| IBS file for 9Meg Burst ( GS88xxxCx )
| DQ driver is programmable
| VDD or VDDQ can be either 1.8V or 2.5V or 3.3V
|  Rev 1.0: Creation
[IBIS Ver]   3.2
[File name]   gs88xxxcx.ibs
[File Rev]   1.0
[Date]   08/12/09
[Component]   GS880f18CT
[Manufacturer]   gsi technology
[Package]
| variable   typ   min   max
R_pkg   0.2   0.1   0.5
L_pkg   4nH   2nH   6nH
C_pkg   1.5pF   1pF   2pF
[Pin]   signal_name model_name  R_pin   L_pin   C_pin
 1   NC   NC
 2   NC   NC
 3   NC   NC
 4   VDDQ   POWER
 5   VSS   GND
 6   NC   NC
 7   NC   NC
 8   DQB1   Progbuf1
 9   DQB2   Progbuf1
 10   VSS   GND
 11   VDDQ   POWER
 12   DQB3   Progbuf1
 13   DQB4   Progbuf1
 14   NC   NC
 15   VDD   POWER
 16   NC   NC
 17   VSS   GND
 18   DQB5   Progbuf1
 19   DQB6   Progbuf1
 20   VDDQ   POWER
 21   VSS   GND
 22   DQB7   Progbuf1
 23   DQB8   Progbuf1
 24   DQB9   Progbuf1
 25   NC   NC
 26   VSS   GND
 27   VDDQ   POWER
 28   NC   NC
 29   NC   NC
 30   NC   NC
 31   LBO#   INBUF
 32   A5   INBUF
 33   A4   INBUF
 34   A3   INBUF
 35   A2   INBUF
 36   A1   INBUF
 37   A0   INBUF
 38   NC   NC
 39   NC   NC
 40   VSS   GND
 41   VDD   POWER
 42   NC   NC
 43   A17   INBUF
 44   A10   INBUF
 45   A11   INBUF
 46   A12   INBUF
 47   A13   INBUF
 48   A14   INBUF
 49   A15   INBUF
 50   A16   INBUF
 51   NC   NC
 52   NC   NC
 53   NC   NC
 54   VDDQ   POWER
 55   VSS   GND
 56   DQA6   Progbuf1
 57   NC   NC
 58   DQA1   Progbuf1
 59   DQA2   Progbuf1
 60   VSS   GND
 61   VDDQ   POWER
 62   DQA3   Progbuf1
 63   DQA4   Progbuf1
 64   ZZ   INBUF
 65   VDD   POWER
 66   NC   NC
 67   VSS   GND
 68   DQA5   Progbuf1
 69   DQA6   Progbuf1
 70   VDDQ   POWER
 71   VSS   GND
 72   DQA7   Progbuf1
 73   DQA8   Progbuf1
 74   DQA9   Progbuf1
 75   NC   NC
 76   VSS   GND
 77   VDDQ   POWER
 78   NC   NC
 79   NC   NC
 80   A18   INBUF
 81   A9   INBUF
 82   A8   INBUF
 83   ADV#   INBUF
 84   ADSP#   INBUF
 85   ADSC#   INBUF
 86   G#   INBUF
 87   BW#   INBUF
 88   GW#   INBUF
 89   CK   INBUF
 90   VSS   GND
 91   VDD   POWER
 92   E3#   INBUF
 93   BA#   INBUF
 94   BB#   INBUF
 95   NC   NC
 96   NC   NC
 97   E2   INBUF
 98   E1#   INBUF
 99   A7   INBUF
 100   A6   INBUF
[Component]   GS880f32CT
[Manufacturer]   gsi technology
[Package]
| variable   typ   min   max
R_pkg   0.2   0.1   0.5
L_pkg   4nH   2nH   6nH
C_pkg   1.5pF   1pF   2pF
[Pin]   signal_name model_name  R_pin   L_pin   C_pin
 1   NC   NC
 2   DQC8   Progbuf1
 3   DQC7   Progbuf1
 4   VDDQ   POWER
 5   VSS   GND
 6   DQC6   Progbuf1
 7   DQC5   Progbuf1
 8   DQC4   Progbuf1
 9   DQC3   Progbuf1
 10   VSS   GND
 11   VDDQ   POWER
 12   DQC2   Progbuf1
 13   DQC1   Progbuf1
 14   NC   NC
 15   VDD   POWER
 16   NC   NC
 17   VSS   GND
 18   DQD1   Progbuf1
 19   DQD2   Progbuf1
 20   VDDQ   POWER
 21   VSS   GND
 22   DQD3   Progbuf1
 23   DQD4   Progbuf1
 24   DQD5   Progbuf1
 25   DQD6   Progbuf1
 26   VSS   GND
 27   VDDQ   POWER
 28   DQD7   Progbuf1
 29   DQD8   Progbuf1
 30   NC   NC
 31   LBO#   INBUF
 32   A5   INBUF
 33   A4   INBUF
 34   A3   INBUF
 35   A2   INBUF
 36   A1   INBUF
 37   A0   INBUF
 38   NC   NC
 39   NC   NC
 40   VSS   GND
 41   VDD   POWER
 42   NC   NC
 43   A17   INBUF
 44   A10   INBUF
 45   A11   INBUF
 46   A12   INBUF
 47   A13   INBUF
 48   A14   INBUF
 49   A15   INBUF
 50   A16   INBUF
 51   NC   NC
 52   DQA8   Progbuf1
 53   DQA7   Progbuf1
 54   VDDQ   POWER
 55   VSS   GND
 56   DQA6   Progbuf1
 57   DQA5   Progbuf1
 58   DQA4   Progbuf1
 59   DQA3   Progbuf1
 60   VSS   GND
 61   VDDQ   POWER
 62   DQA2   Progbuf1
 63   DQA1   Progbuf1
 64   ZZ   INBUF
 65   VDD   POWER
 66   NC   NC
 67   VSS   GND
 68   DQB1   Progbuf1
 69   DQB2   Progbuf1
 70   VDDQ   POWER
 71   VSS   GND
 72   DQB3   Progbuf1
 73   DQB4   Progbuf1
 74   DQB5   Progbuf1
 75   DQB6   Progbuf1
 76   VSS   GND
 77   VDDQ   POWER
 78   DQB7   Progbuf1
 79   DQB8   Progbuf1
 80   NC   NC
 81   A9   INBUF
 82   A8   INBUF
 83   ADV#   INBUF
 84   ADSP#   INBUF
 85   ADSC#   INBUF
 86   G#   INBUF
 87   BW#   INBUF
 88   GW#   INBUF
 89   CK   INBUF
 90   VSS   GND
 91   VDD   POWER
 92   E3#   INBUF
 93   BA#   INBUF
 94   BB#   INBUF
 95   BC#   INBUF
 96   BD#   INBUF
 97   E2   INBUF
 98   E1#   INBUF
 99   A7   INBUF
 100   A6   INBUF
[Component]   GS880f36CT
[Manufacturer]   gsi technology
[Package]
| variable   typ   min   max
R_pkg   0.2   0.1   0.5
L_pkg   4nH   2nH   6nH
C_pkg   1.5pF   1pF   2pF
[Pin]   signal_name model_name  R_pin   L_pin   C_pin
 1   DQC9   Progbuf1
 2   DQC8   Progbuf1
 3   DQC7   Progbuf1
 4   VDDQ   POWER
 5   VSS   GND
 6   DQC6   Progbuf1
 7   DQC5   Progbuf1
 8   DQC4   Progbuf1
 9   DQC3   Progbuf1
 10   VSS   GND
 11   VDDQ   POWER
 12   DQC2   Progbuf1
 13   DQC1   Progbuf1
 14   NC   NC
 15   VDD   POWER
 16   NC   NC
 17   VSS   GND
 18   DQD1   Progbuf1
 19   DQD2   Progbuf1
 20   VDDQ   POWER
 21   VSS   GND
 22   DQD3   Progbuf1
 23   DQD4   Progbuf1
 24   DQD5   Progbuf1
 25   DQD6   Progbuf1
 26   VSS   GND
 27   VDDQ   POWER
 28   DQD7   Progbuf1
 29   DQD8   Progbuf1
 30   DQD9   Progbuf1
 31   LBO#   INBUF
 32   A5   INBUF
 33   A4   INBUF
 34   A3   INBUF
 35   A2   INBUF
 36   A1   INBUF
 37   A0   INBUF
 38   NC   NC
 39   NC   NC
 40   VSS   GND
 41   VDD   POWER
 42   A18   INBUF
 43   A17   INBUF
 44   A10   INBUF
 45   A11   INBUF
 46   A12   INBUF
 47   A13   INBUF
 48   A14   INBUF
 49   A15   INBUF
 50   A16   INBUF
 51   DQA9   Progbuf1
 52   DQA8   Progbuf1
 53   DQA7   Progbuf1
 54   VDDQ   POWER
 55   VSS   GND
 56   DQA6   Progbuf1
 57   DQA5   Progbuf1
 58   DQA4   Progbuf1
 59   DQA3   Progbuf1
 60   VSS   GND
 61   VDDQ   POWER
 62   DQA2   Progbuf1
 63   DQA1   Progbuf1
 64   ZZ   INBUF
 65   VDD   POWER
 66   NC   NC
 67   VSS   GND
 68   DQB1   Progbuf1
 69   DQB2   Progbuf1
 70   VDDQ   POWER
 71   VSS   GND
 72   DQB3   Progbuf1
 73   DQB4   Progbuf1
 74   DQB5   Progbuf1
 75   DQB6   Progbuf1
 76   VSS   GND
 77   VDDQ   POWER
 78   DQB7   Progbuf1
 79   DQB8   Progbuf1
 80   DQB9   Progbuf1
 81   A9   INBUF
 82   A8   INBUF
 83   ADV#   INBUF
 84   ADSP#   INBUF
 85   ADSC#   INBUF
 86   G#   INBUF
 87   BW#   INBUF
 88   GW#   INBUF
 89   CK   INBUF
 90   VSS   GND
 91   VDD   POWER
 92   E3#   INBUF
 93   BA#   INBUF
 94   BB#   INBUF
 95   BC#   INBUF
 96   BD#   INBUF
 97   E2   INBUF
 98   E1#   INBUF
 99   A7   INBUF
 100   A6   INBUF
[Component]   GS880L18CT
[Manufacturer]   gsi technology
[Package]
| variable   typ   min   max
R_pkg   0.2   0.1   0.5
L_pkg   4nH   2nH   6nH
C_pkg   1.5pF   1pF   2pF
[Pin]   signal_name model_name  R_pin   L_pin   C_pin
 1   NC   NC
 2   NC   NC
 3   NC   NC
 4   VDDQ   POWER
 5   VSS   GND
 6   NC   NC
 7   NC   NC
 8   DQB1   Progbuf1
 9   DQB2   Progbuf1
 10   VSS   GND
 11   VDDQ   POWER
 12   DQB3   Progbuf1
 13   DQB4   Progbuf1
 14   FT#   INBUF
 15   VDD   POWER
 16   NC   NC
 17   VSS   GND
 18   DQB5   Progbuf1
 19   DQB6   Progbuf1
 20   VDDQ   POWER
 21   VSS   GND
 22   DQB7   Progbuf1
 23   DQB8   Progbuf1
 24   DQB9   Progbuf1
 25   NC   NC
 26   VSS   GND
 27   VDDQ   POWER
 28   NC   NC
 29   NC   NC
 30   NC   NC
 31   LBO#   INBUF
 32   A5   INBUF
 33   A4   INBUF
 34   A3   INBUF
 35   A2   INBUF
 36   A1   INBUF
 37   A0   INBUF
 38   NC   NC
 39   NC   NC
 40   VSS   GND
 41   VDD   POWER
 42   NC   NC
 43   A17   INBUF
 44   A10   INBUF
 45   A11   INBUF
 46   A12   INBUF
 47   A13   INBUF
 48   A14   INBUF
 49   A15   INBUF
 50   A16   INBUF
 51   NC   NC
 52   NC   NC
 53   NC   NC
 54   VDDQ   POWER
 55   VSS   GND
 56   DQA6   Progbuf1
 57   NC   NC
 58   DQA1   Progbuf1
 59   DQA2   Progbuf1
 60   VSS   GND
 61   VDDQ   POWER
 62   DQA3   Progbuf1
 63   DQA4   Progbuf1
 64   ZZ   INBUF
 65   VDD   POWER
 66   NC   NC
 67   VSS   GND
 68   DQA5   Progbuf1
 69   DQA6   Progbuf1
 70   VDDQ   POWER
 71   VSS   GND
 72   DQA7   Progbuf1
 73   DQA8   Progbuf1
 74   DQA9   Progbuf1
 75   NC   NC
 76   VSS   GND
 77   VDDQ   POWER
 78   NC   NC
 79   NC   NC
 80   A18   INBUF
 81   A9   INBUF
 82   A8   INBUF
 83   ADV#   INBUF
 84   ADSP#   INBUF
 85   ADSC#   INBUF
 86   G#   INBUF
 87   BW#   INBUF
 88   GW#   INBUF
 89   CK   INBUF
 90   VSS   GND
 91   VDD   POWER
 92   E3#   INBUF
 93   BA#   INBUF
 94   BB#   INBUF
 95   NC   NC
 96   NC   NC
 97   E2   INBUF
 98   E1#   INBUF
 99   A7   INBUF
 100   A6   INBUF
[Component]   GS880l32CT
[Manufacturer]   gsi technology
[Package]
| variable   typ   min   max
R_pkg   0.2   0.1   0.5
L_pkg   4nH   2nH   6nH
C_pkg   1.5pF   1pF   2pF
[Pin]   signal_name model_name  R_pin   L_pin   C_pin
 1   NC   NC
 2   DQC8   Progbuf1
 3   DQC7   Progbuf1
 4   VDDQ   POWER
 5   VSS   GND
 6   DQC6   Progbuf1
 7   DQC5   Progbuf1
 8   DQC4   Progbuf1
 9   DQC3   Progbuf1
 10   VSS   GND
 11   VDDQ   POWER
 12   DQC2   Progbuf1
 13   DQC1   Progbuf1
 14   FT#   INBUF
 15   VDD   POWER
 16   NC   NC
 17   VSS   GND
 18   DQD1   Progbuf1
 19   DQD2   Progbuf1
 20   VDDQ   POWER
 21   VSS   GND
 22   DQD3   Progbuf1
 23   DQD4   Progbuf1
 24   DQD5   Progbuf1
 25   DQD6   Progbuf1
 26   VSS   GND
 27   VDDQ   POWER
 28   DQD7   Progbuf1
 29   DQD8   Progbuf1
 30   NC   NC
 31   LBO#   INBUF
 32   A5   INBUF
 33   A4   INBUF
 34   A3   INBUF
 35   A2   INBUF
 36   A1   INBUF
 37   A0   INBUF
 38   NC   NC
 39   NC   NC
 40   VSS   GND
 41   VDD   POWER
 42   NC   NC
 43   A17   INBUF
 44   A10   INBUF
 45   A11   INBUF
 46   A12   INBUF
 47   A13   INBUF
 48   A14   INBUF
 49   A15   INBUF
 50   A16   INBUF
 51   NC   NC
 52   DQA8   Progbuf1
 53   DQA7   Progbuf1
 54   VDDQ   POWER
 55   VSS   GND
 56   DQA6   Progbuf1
 57   DQA5   Progbuf1
 58   DQA4   Progbuf1
 59   DQA3   Progbuf1
 60   VSS   GND
 61   VDDQ   POWER
 62   DQA2   Progbuf1
 63   DQA1   Progbuf1
 64   ZZ   INBUF
 65   VDD   POWER
 66   NC   NC
 67   VSS   GND
 68   DQB1   Progbuf1
 69   DQB2   Progbuf1
 70   VDDQ   POWER
 71   VSS   GND
 72   DQB3   Progbuf1
 73   DQB4   Progbuf1
 74   DQB5   Progbuf1
 75   DQB6   Progbuf1
 76   VSS   GND
 77   VDDQ   POWER
 78   DQB7   Progbuf1
 79   DQB8   Progbuf1
 80   NC   NC
 81   A9   INBUF
 82   A8   INBUF
 83   ADV#   INBUF
 84   ADSP#   INBUF
 85   ADSC#   INBUF
 86   G#   INBUF
 87   BW#   INBUF
 88   GW#   INBUF
 89   CK   INBUF
 90   VSS   GND
 91   VDD   POWER
 92   E3#   INBUF
 93   BA#   INBUF
 94   BB#   INBUF
 95   BC#   INBUF
 96   BD#   INBUF
 97   E2   INBUF
 98   E1#   INBUF
 99   A7   INBUF
 100   A6   INBUF
[Component]   GS880L36CT
[Manufacturer]   gsi technology
[Package]
| variable   typ   min   max
R_pkg   0.2   0.1   0.5
L_pkg   4nH   2nH   6nH
C_pkg   1.5pF   1pF   2pF
[Pin]   signal_name model_name  R_pin   L_pin   C_pin
 1   DQC9   Progbuf1
 2   DQC8   Progbuf1
 3   DQC7   Progbuf1
 4   VDDQ   POWER
 5   VSS   GND
 6   DQC6   Progbuf1
 7   DQC5   Progbuf1
 8   DQC4   Progbuf1
 9   DQC3   Progbuf1
 10   VSS   GND
 11   VDDQ   POWER
 12   DQC2   Progbuf1
 13   DQC1   Progbuf1
 14   FT#   INBUF
 15   VDD   POWER
 16   NC   NC
 17   VSS   GND
 18   DQD1   Progbuf1
 19   DQD2   Progbuf1
 20   VDDQ   POWER
 21   VSS   GND
 22   DQD3   Progbuf1
 23   DQD4   Progbuf1
 24   DQD5   Progbuf1
 25   DQD6   Progbuf1
 26   VSS   GND
 27   VDDQ   POWER
 28   DQD7   Progbuf1
 29   DQD8   Progbuf1
 30   DQD9   Progbuf1
 31   LBO#   INBUF
 32   A5   INBUF
 33   A4   INBUF
 34   A3   INBUF
 35   A2   INBUF
 36   A1   INBUF
 37   A0   INBUF
 38   NC   NC
 39   NC   NC
 40   VSS   GND
 41   VDD   POWER
 42   A18   INBUF
 43   A17   INBUF
 44   A10   INBUF
 45   A11   INBUF
 46   A12   INBUF
 47   A13   INBUF
 48   A14   INBUF
 49   A15   INBUF
 50   A16   INBUF
 51   DQA9   Progbuf1
 52   DQA8   Progbuf1
 53   DQA7   Progbuf1
 54   VDDQ   POWER
 55   VSS   GND
 56   DQA6   Progbuf1
 57   DQA5   Progbuf1
 58   DQA4   Progbuf1
 59   DQA3   Progbuf1
 60   VSS   GND
 61   VDDQ   POWER
 62   DQA2   Progbuf1
 63   DQA1   Progbuf1
 64   ZZ   INBUF
 65   VDD   POWER
 66   NC   NC
 67   VSS   GND
 68   DQB1   Progbuf1
 69   DQB2   Progbuf1
 70   VDDQ   POWER
 71   VSS   GND
 72   DQB3   Progbuf1
 73   DQB4   Progbuf1
 74   DQB5   Progbuf1
 75   DQB6   Progbuf1
 76   VSS   GND
 77   VDDQ   POWER
 78   DQB7   Progbuf1
 79   DQB8   Progbuf1
 80   DQB9   Progbuf1
 81   A9   INBUF
 82   A8   INBUF
 83   ADV#   INBUF
 84   ADSP#   INBUF
 85   ADSC#   INBUF
 86   G#   INBUF
 87   BW#   INBUF
 88   GW#   INBUF
 89   CK   INBUF
 90   VSS   GND
 91   VDD   POWER
 92   E3#   INBUF
 93   BA#   INBUF
 94   BB#   INBUF
 95   BC#   INBUF
 96   BD#   INBUF
 97   E2   INBUF
 98   E1#   INBUF
 99   A7   INBUF
 100   A6   INBUF
[Component]   GS88018CT
[Manufacturer]   gsi technology
[Package]
| variable   typ   min   max
R_pkg   0.2   0.1   0.5
L_pkg   4nH   2nH   6nH
C_pkg   1.5pF   1pF   2pF
[Pin]   signal_name model_name  R_pin   L_pin   C_pin
 1   NC   NC
 2   NC   NC
 3   NC   NC
 4   VDDQ   POWER
 5   VSS   GND
 6   NC   NC
 7   NC   NC
 8   DQB1   Progbuf1
 9   DQB2   Progbuf1
 10   VSS   GND
 11   VDDQ   POWER
 12   DQB3   Progbuf1
 13   DQB4   Progbuf1
 14   FT#   INBUF
 15   VDD   POWER
 16   NC   NC
 17   VSS   GND
 18   DQB5   Progbuf1
 19   DQB6   Progbuf1
 20   VDDQ   POWER
 21   VSS   GND
 22   DQB7   Progbuf1
 23   DQB8   Progbuf1
 24   DQB9   Progbuf1
 25   NC   NC
 26   VSS   GND
 27   VDDQ   POWER
 28   NC   NC
 29   NC   NC
 30   NC   NC
 31   LBO#   INBUF
 32   A5   INBUF
 33   A4   INBUF
 34   A3   INBUF
 35   A2   INBUF
 36   A1   INBUF
 37   A0   INBUF
 38   NC   NC
 39   NC   NC
 40   VSS   GND
 41   VDD   POWER
 42   NC   NC
 43   A17   INBUF
 44   A10   INBUF
 45   A11   INBUF
 46   A12   INBUF
 47   A13   INBUF
 48   A14   INBUF
 49   A15   INBUF
 50   A16   INBUF
 51   NC   NC
 52   NC   NC
 53   NC   NC
 54   VDDQ   POWER
 55   VSS   GND
 56   DQA6   Progbuf1
 57   NC   NC
 58   DQA1   Progbuf1
 59   DQA2   Progbuf1
 60   VSS   GND
 61   VDDQ   POWER
 62   DQA3   Progbuf1
 63   DQA4   Progbuf1
 64   ZZ   INBUF
 65   VDD   POWER
 66   NC   NC
 67   VSS   GND
 68   DQA5   Progbuf1
 69   DQA6   Progbuf1
 70   VDDQ   POWER
 71   VSS   GND
 72   DQA7   Progbuf1
 73   DQA8   Progbuf1
 74   DQA9   Progbuf1
 75   NC   NC
 76   VSS   GND
 77   VDDQ   POWER
 78   NC   NC
 79   NC   NC
 80   A18   INBUF
 81   A9   INBUF
 82   A8   INBUF
 83   ADV#   INBUF
 84   ADSP#   INBUF
 85   ADSC#   INBUF
 86   G#   INBUF
 87   BW#   INBUF
 88   GW#   INBUF
 89   CK   INBUF
 90   VSS   GND
 91   VDD   POWER
 92   E3#   INBUF
 93   BA#   INBUF
 94   BB#   INBUF
 95   NC   NC
 96   NC   NC
 97   E2   INBUF
 98   E1#   INBUF
 99   A7   INBUF
 100   A6   INBUF
[Component]   GS88019CT
[Manufacturer]   gsi technology
[Package]
| variable   typ   min   max
R_pkg   0.2   0.1   0.5
L_pkg   4nH   2nH   6nH
C_pkg   1.5pF   1pF   2pF
[Pin]   signal_name model_name  R_pin   L_pin   C_pin
 1   NC   NC
 2   NC   NC
 3   NC   NC
 4   VDDQ   POWER
 5   VSS   GND
 6   NC   NC
 7   NC   NC
 8   DQB1   Progbuf1
 9   DQB2   Progbuf1
 10   VSS   GND
 11   VDDQ   POWER
 12   DQB3   Progbuf1
 13   DQB4   Progbuf1
 14   FT#   INBUF
 15   VDD   POWER
 16   NC   NC
 17   VSS   GND
 18   DQB5   Progbuf1
 19   DQB6   Progbuf1
 20   VDDQ   POWER
 21   VSS   GND
 22   DQB7   Progbuf1
 23   DQB8   Progbuf1
 24   DQB9   Progbuf1
 25   NC   NC
 26   VSS   GND
 27   VDDQ   POWER
 28   NC   NC
 29   NC   NC
 30   NC   NC
 31   LBO#   INBUF
 32   A5   INBUF
 33   A4   INBUF
 34   A3   INBUF
 35   A2   INBUF
 36   A1   INBUF
 37   A0   INBUF
 38   NC   NC
 39   NC   NC
 40   VSS   GND
 41   VDD   POWER
 42   NC   NC
 43   A17   INBUF
 44   A10   INBUF
 45   A11   INBUF
 46   A12   INBUF
 47   A13   INBUF
 48   A14   INBUF
 49   A15   INBUF
 50   A16   INBUF
 51   NC   NC
 52   NC   NC
 53   NC   NC
 54   VDDQ   POWER
 55   VSS   GND
 56   DQA6   Progbuf1
 57   NC   NC
 58   DQA1   Progbuf1
 59   DQA2   Progbuf1
 60   VSS   GND
 61   VDDQ   POWER
 62   DQA3   Progbuf1
 63   DQA4   Progbuf1
 64   ZZ   INBUF
 65   VDD   POWER
 66   NC   NC
 67   VSS   GND
 68   DQA5   Progbuf1
 69   DQA6   Progbuf1
 70   VDDQ   POWER
 71   VSS   GND
 72   DQA7   Progbuf1
 73   DQA8   Progbuf1
 74   DQA9   Progbuf1
 75   NC   NC
 76   VSS   GND
 77   VDDQ   POWER
 78   NC   NC
 79   NC   NC
 80   A18   INBUF
 81   A9   INBUF
 82   A8   INBUF
 83   ADV#   INBUF
 84   ADSP#   INBUF
 85   ADSC#   INBUF
 86   G#   INBUF
 87   BW#   INBUF
 88   GW#   INBUF
 89   CK   INBUF
 90   VSS   GND
 91   VDD   POWER
 92   E3#   INBUF
 93   BA#   INBUF
 94   BB#   INBUF
 95   NC   NC
 96   NC   NC
 97   E2   INBUF
 98   E1#   INBUF
 99   A7   INBUF
 100   A6   INBUF
[Component]   GS88032CT
[Manufacturer]   gsi technology
[Package]
| variable   typ   min   max
R_pkg   0.2   0.1   0.5
L_pkg   4nH   2nH   6nH
C_pkg   1.5pF   1pF   2pF
[Pin]   signal_name model_name  R_pin   L_pin   C_pin
 1   NC   NC
 2   DQC8   Progbuf1
 3   DQC7   Progbuf1
 4   VDDQ   POWER
 5   VSS   GND
 6   DQC6   Progbuf1
 7   DQC5   Progbuf1
 8   DQC4   Progbuf1
 9   DQC3   Progbuf1
 10   VSS   GND
 11   VDDQ   POWER
 12   DQC2   Progbuf1
 13   DQC1   Progbuf1
 14   FT#   INBUF
 15   VDD   POWER
 16   NC   NC
 17   VSS   GND
 18   DQD1   Progbuf1
 19   DQD2   Progbuf1
 20   VDDQ   POWER
 21   VSS   GND
 22   DQD3   Progbuf1
 23   DQD4   Progbuf1
 24   DQD5   Progbuf1
 25   DQD6   Progbuf1
 26   VSS   GND
 27   VDDQ   POWER
 28   DQD7   Progbuf1
 29   DQD8   Progbuf1
 30   NC   NC
 31   LBO#   INBUF
 32   A5   INBUF
 33   A4   INBUF
 34   A3   INBUF
 35   A2   INBUF
 36   A1   INBUF
 37   A0   INBUF
 38   NC   NC
 39   NC   NC
 40   VSS   GND
 41   VDD   POWER
 42   NC   NC
 43   A17   INBUF
 44   A10   INBUF
 45   A11   INBUF
 46   A12   INBUF
 47   A13   INBUF
 48   A14   INBUF
 49   A15   INBUF
 50   A16   INBUF
 51   NC   NC
 52   DQA8   Progbuf1
 53   DQA7   Progbuf1
 54   VDDQ   POWER
 55   VSS   GND
 56   DQA6   Progbuf1
 57   DQA5   Progbuf1
 58   DQA4   Progbuf1
 59   DQA3   Progbuf1
 60   VSS   GND
 61   VDDQ   POWER
 62   DQA2   Progbuf1
 63   DQA1   Progbuf1
 64   ZZ   INBUF
 65   VDD   POWER
 66   NC   NC
 67   VSS   GND
 68   DQB1   Progbuf1
 69   DQB2   Progbuf1
 70   VDDQ   POWER
 71   VSS   GND
 72   DQB3   Progbuf1
 73   DQB4   Progbuf1
 74   DQB5   Progbuf1
 75   DQB6   Progbuf1
 76   VSS   GND
 77   VDDQ   POWER
 78   DQB7   Progbuf1
 79   DQB8   Progbuf1
 80   NC   NC
 81   A9   INBUF
 82   A8   INBUF
 83   ADV#   INBUF
 84   ADSP#   INBUF
 85   ADSC#   INBUF
 86   G#   INBUF
 87   BW#   INBUF
 88   GW#   INBUF
 89   CK   INBUF
 90   VSS   GND
 91   VDD   POWER
 92   E3#   INBUF
 93   BA#   INBUF
 94   BB#   INBUF
 95   BC#   INBUF
 96   BD#   INBUF
 97   E2   INBUF
 98   E1#   INBUF
 99   A7   INBUF
 100   A6   INBUF
[Component]   GS88033CT
[Manufacturer]   gsi technology
[Package]
| variable   typ   min   max
R_pkg   0.2   0.1   0.5
L_pkg   4nH   2nH   6nH
C_pkg   1.5pF   1pF   2pF
[Pin]   signal_name model_name  R_pin   L_pin   C_pin
 1   NC   NC
 2   DQC8   Progbuf1
 3   DQC7   Progbuf1
 4   VDDQ   POWER
 5   VSS   GND
 6   DQC6   Progbuf1
 7   DQC5   Progbuf1
 8   DQC4   Progbuf1
 9   DQC3   Progbuf1
 10   VSS   GND
 11   VDDQ   POWER
 12   DQC2   Progbuf1
 13   DQC1   Progbuf1
 14   FT#   INBUF
 15   VDD   POWER
 16   NC   NC
 17   VSS   GND
 18   DQD1   Progbuf1
 19   DQD2   Progbuf1
 20   VDDQ   POWER
 21   VSS   GND
 22   DQD3   Progbuf1
 23   DQD4   Progbuf1
 24   DQD5   Progbuf1
 25   DQD6   Progbuf1
 26   VSS   GND
 27   VDDQ   POWER
 28   DQD7   Progbuf1
 29   DQD8   Progbuf1
 30   NC   NC
 31   LBO#   INBUF
 32   A5   INBUF
 33   A4   INBUF
 34   A3   INBUF
 35   A2   INBUF
 36   A1   INBUF
 37   A0   INBUF
 38   NC   NC
 39   NC   NC
 40   VSS   GND
 41   VDD   POWER
 42   NC   NC
 43   A17   INBUF
 44   A10   INBUF
 45   A11   INBUF
 46   A12   INBUF
 47   A13   INBUF
 48   A14   INBUF
 49   A15   INBUF
 50   A16   INBUF
 51   NC   NC
 52   DQA8   Progbuf1
 53   DQA7   Progbuf1
 54   VDDQ   POWER
 55   VSS   GND
 56   DQA6   Progbuf1
 57   DQA5   Progbuf1
 58   DQA4   Progbuf1
 59   DQA3   Progbuf1
 60   VSS   GND
 61   VDDQ   POWER
 62   DQA2   Progbuf1
 63   DQA1   Progbuf1
 64   ZZ   INBUF
 65   VDD   POWER
 66   NC   NC
 67   VSS   GND
 68   DQB1   Progbuf1
 69   DQB2   Progbuf1
 70   VDDQ   POWER
 71   VSS   GND
 72   DQB3   Progbuf1
 73   DQB4   Progbuf1
 74   DQB5   Progbuf1
 75   DQB6   Progbuf1
 76   VSS   GND
 77   VDDQ   POWER
 78   DQB7   Progbuf1
 79   DQB8   Progbuf1
 80   NC   NC
 81   A9   INBUF
 82   A8   INBUF
 83   ADV#   INBUF
 84   ADSP#   INBUF
 85   ADSC#   INBUF
 86   G#   INBUF
 87   BW#   INBUF
 88   GW#   INBUF
 89   CK   INBUF
 90   VSS   GND
 91   VDD   POWER
 92   E3#   INBUF
 93   BA#   INBUF
 94   BB#   INBUF
 95   BC#   INBUF
 96   BD#   INBUF
 97   E2   INBUF
 98   E1#   INBUF
 99   A7   INBUF
 100   A6   INBUF
[Component]   GS88036CT
[Manufacturer]   gsi technology
[Package]
| variable   typ   min   max
R_pkg   0.2   0.1   0.5
L_pkg   4nH   2nH   6nH
C_pkg   1.5pF   1pF   2pF
[Pin]   signal_name model_name  R_pin   L_pin   C_pin
 1   DQC9   Progbuf1
 2   DQC8   Progbuf1
 3   DQC7   Progbuf1
 4   VDDQ   POWER
 5   VSS   GND
 6   DQC6   Progbuf1
 7   DQC5   Progbuf1
 8   DQC4   Progbuf1
 9   DQC3   Progbuf1
 10   VSS   GND
 11   VDDQ   POWER
 12   DQC2   Progbuf1
 13   DQC1   Progbuf1
 14   FT#   INBUF
 15   VDD   POWER
 16   NC   NC
 17   VSS   GND
 18   DQD1   Progbuf1
 19   DQD2   Progbuf1
 20   VDDQ   POWER
 21   VSS   GND
 22   DQD3   Progbuf1
 23   DQD4   Progbuf1
 24   DQD5   Progbuf1
 25   DQD6   Progbuf1
 26   VSS   GND
 27   VDDQ   POWER
 28   DQD7   Progbuf1
 29   DQD8   Progbuf1
 30   DQD9   Progbuf1
 31   LBO#   INBUF
 32   A5   INBUF
 33   A4   INBUF
 34   A3   INBUF
 35   A2   INBUF
 36   A1   INBUF
 37   A0   INBUF
 38   NC   NC
 39   NC   NC
 40   VSS   GND
 41   VDD   POWER
 42   A18   INBUF
 43   A17   INBUF
 44   A10   INBUF
 45   A11   INBUF
 46   A12   INBUF
 47   A13   INBUF
 48   A14   INBUF
 49   A15   INBUF
 50   A16   INBUF
 51   DQA9   Progbuf1
 52   DQA8   Progbuf1
 53   DQA7   Progbuf1
 54   VDDQ   POWER
 55   VSS   GND
 56   DQA6   Progbuf1
 57   DQA5   Progbuf1
 58   DQA4   Progbuf1
 59   DQA3   Progbuf1
 60   VSS   GND
 61   VDDQ   POWER
 62   DQA2   Progbuf1
 63   DQA1   Progbuf1
 64   ZZ   INBUF
 65   VDD   POWER
 66   NC   NC
 67   VSS   GND
 68   DQB1   Progbuf1
 69   DQB2   Progbuf1
 70   VDDQ   POWER
 71   VSS   GND
 72   DQB3   Progbuf1
 73   DQB4   Progbuf1
 74   DQB5   Progbuf1
 75   DQB6   Progbuf1
 76   VSS   GND
 77   VDDQ   POWER
 78   DQB7   Progbuf1
 79   DQB8   Progbuf1
 80   DQB9   Progbuf1
 81   A9   INBUF
 82   A8   INBUF
 83   ADV#   INBUF
 84   ADSP#   INBUF
 85   ADSC#   INBUF
 86   G#   INBUF
 87   BW#   INBUF
 88   GW#   INBUF
 89   CK   INBUF
 90   VSS   GND
 91   VDD   POWER
 92   E3#   INBUF
 93   BA#   INBUF
 94   BB#   INBUF
 95   BC#   INBUF
 96   BD#   INBUF
 97   E2   INBUF
 98   E1#   INBUF
 99   A7   INBUF
 100   A6   INBUF
[Component]   GS88037CT
[Manufacturer]   gsi technology
[Package]
| variable   typ   min   max
R_pkg   0.2   0.1   0.5
L_pkg   4nH   2nH   6nH
C_pkg   1.5pF   1pF   2pF
[Pin]   signal_name model_name  R_pin   L_pin   C_pin
 1   DQC9   Progbuf1
 2   DQC8   Progbuf1
 3   DQC7   Progbuf1
 4   VDDQ   POWER
 5   VSS   GND
 6   DQC6   Progbuf1
 7   DQC5   Progbuf1
 8   DQC4   Progbuf1
 9   DQC3   Progbuf1
 10   VSS   GND
 11   VDDQ   POWER
 12   DQC2   Progbuf1
 13   DQC1   Progbuf1
 14   FT#   INBUF
 15   VDD   POWER
 16   NC   NC
 17   VSS   GND
 18   DQD1   Progbuf1
 19   DQD2   Progbuf1
 20   VDDQ   POWER
 21   VSS   GND
 22   DQD3   Progbuf1
 23   DQD4   Progbuf1
 24   DQD5   Progbuf1
 25   DQD6   Progbuf1
 26   VSS   GND
 27   VDDQ   POWER
 28   DQD7   Progbuf1
 29   DQD8   Progbuf1
 30   DQD9   Progbuf1
 31   LBO#   INBUF
 32   A5   INBUF
 33   A4   INBUF
 34   A3   INBUF
 35   A2   INBUF
 36   A1   INBUF
 37   A0   INBUF
 38   NC   NC
 39   NC   NC
 40   VSS   GND
 41   VDD   POWER
 42   A18   INBUF
 43   A17   INBUF
 44   A10   INBUF
 45   A11   INBUF
 46   A12   INBUF
 47   A13   INBUF
 48   A14   INBUF
 49   A15   INBUF
 50   A16   INBUF
 51   DQA9   Progbuf1
 52   DQA8   Progbuf1
 53   DQA7   Progbuf1
 54   VDDQ   POWER
 55   VSS   GND
 56   DQA6   Progbuf1
 57   DQA5   Progbuf1
 58   DQA4   Progbuf1
 59   DQA3   Progbuf1
 60   VSS   GND
 61   VDDQ   POWER
 62   DQA2   Progbuf1
 63   DQA1   Progbuf1
 64   ZZ   INBUF
 65   VDD   POWER
 66   NC   NC
 67   VSS   GND
 68   DQB1   Progbuf1
 69   DQB2   Progbuf1
 70   VDDQ   POWER
 71   VSS   GND
 72   DQB3   Progbuf1
 73   DQB4   Progbuf1
 74   DQB5   Progbuf1
 75   DQB6   Progbuf1
 76   VSS   GND
 77   VDDQ   POWER
 78   DQB7   Progbuf1
 79   DQB8   Progbuf1
 80   DQB9   Progbuf1
 81   A9   INBUF
 82   A8   INBUF
 83   ADV#   INBUF
 84   ADSP#   INBUF
 85   ADSC#   INBUF
 86   G#   INBUF
 87   BW#   INBUF
 88   GW#   INBUF
 89   CK   INBUF
 90   VSS   GND
 91   VDD   POWER
 92   E3#   INBUF
 93   BA#   INBUF
 94   BB#   INBUF
 95   BC#   INBUF
 96   BD#   INBUF
 97   E2   INBUF
 98   E1#   INBUF
 99   A7   INBUF
 100   A6   INBUF
[Component]   GS881E18CT
[Manufacturer]   gsi technology
[Package]
| variable   typ   min   max
R_pkg   0.2   0.1   0.5
L_pkg   4nH   2nH   6nH
C_pkg   1.5pF   1pF   2pF
[Pin]   signal_name model_name  R_pin   L_pin   C_pin
 1   NC   NC
 2   NC   NC
 3   NC   NC
 4   VDDQ   POWER
 5   VSS   GND
 6   NC   NC
 7   NC   NC
 8   DQB1   Progbuf1
 9   DQB2   Progbuf1
 10   VSS   GND
 11   VDDQ   POWER
 12   DQB3   Progbuf1
 13   DQB4   Progbuf1
 14   FT#   INBUF
 15   VDD   POWER
 16   NC   NC
 17   VSS   GND
 18   DQB5   Progbuf1
 19   DQB6   Progbuf1
 20   VDDQ   POWER
 21   VSS   GND
 22   DQB7   Progbuf1
 23   DQB8   Progbuf1
 24   DQB9   Progbuf1
 25   NC   NC
 26   VSS   GND
 27   VDDQ   POWER
 28   NC   NC
 29   NC   NC
 30   NC   NC
 31   LBO#   INBUF
 32   A5   INBUF
 33   A4   INBUF
 34   A3   INBUF
 35   A2   INBUF
 36   A1   INBUF
 37   A0   INBUF
 38   TMS   INBUF
 39   TDI   INBUF
 40   VSS   GND
 41   VDD   POWER
 42   TDO   Progbuf2
 43   TCK   INBUF
 44   A10   INBUF
 45   A11   INBUF
 46   A12   INBUF
 47   A13   INBUF
 48   A14   INBUF
 49   A15   INBUF
 50   A16   INBUF
 51   NC   NC
 52   NC   NC
 53   NC   NC
 54   VDDQ   POWER
 55   VSS   GND
 56   DQA6   Progbuf1
 57   NC   NC
 58   DQA1   Progbuf1
 59   DQA2   Progbuf1
 60   VSS   GND
 61   VDDQ   POWER
 62   DQA3   Progbuf1
 63   DQA4   Progbuf1
 64   ZZ   INBUF
 65   VDD   POWER
 66   NC   NC
 67   VSS   GND
 68   DQA5   Progbuf1
 69   DQA6   Progbuf1
 70   VDDQ   POWER
 71   VSS   GND
 72   DQA7   Progbuf1
 73   DQA8   Progbuf1
 74   DQA9   Progbuf1
 75   NC   NC
 76   VSS   GND
 77   VDDQ   POWER
 78   NC   NC
 79   NC   NC
 80   A18   INBUF
 81   A9   INBUF
 82   A8   INBUF
 83   ADV#   INBUF
 84   ADSP#   INBUF
 85   ADSC#   INBUF
 86   G#   INBUF
 87   BW#   INBUF
 88   GW#   INBUF
 89   CK   INBUF
 90   VSS   GND
 91   VDD   POWER
 92   A17   INBUF
 93   BA#   INBUF
 94   BB#   INBUF
 95   NC   NC
 96   NC   NC
 97   NC   NC
 98   E1#   INBUF
 99   A7   INBUF
 100   A6   INBUF
[Component]   GS881E18CD
[Manufacturer]   gsi technology
[Package]
| variable   typ   min   max
R_pkg   0.2   0.1   0.5
L_pkg   3nH   1nH   5nH
C_pkg   1.5pF   1pF   3pF
[Pin]   signal_name model_name  R_pin   L_pin   C_pin
 A1   VDDQ   POWER
 A2   A6   INBUF
 A3   A7   INBUF
 A4   ADSP#   INBUF
 A5   A8   INBUF
 A6   A9   INBUF
 A7   VDDQ   POWER
 B1   NC   NC
 B2   NC   NC
 B3   A4   INBUF
 B4   ADSC#   INBUF
 B5   A15   INBUF
 B6   A17   INBUF
 B7   NC   NC
 C1   NC   NC
 C2   A5   INBUF
 C3   A3   INBUF
 C4   VDD   POWER
 C5   A14   INBUF
 C6   A16   INBUF
 C7   NC   NC
 D1   DQB1   Progbuf1
 D2   NC   NC
 D3   VSS   GND
 D4   NC   NC
 D5   VSS   GND
 D6   DQA9   Progbuf1
 D7   NC   NC
 E1   NC   NC
 E2   DQB2   Progbuf1
 E3   VSS   GND
 E4   E1#   INBUF
 E5   VSS   GND
 E6   NC   NC
 E7   DQA8   Progbuf1
 F1   VDDQ   POWER
 F2   NC   NC
 F3   VSS   GND
 F4   G#   INBUF
 F5   VSS   GND
 F6   DQA7   Progbuf1
 F7   VDDQ   POWER
 G1   NC   NC
 G2   DQB3   Progbuf1
 G3   BB#   INBUF
 G4   ADV#   INBUF
 G5   NC   NC
 G6   NC   NC
 G7   DQA6   Progbuf1
 H1   DQB4   Progbuf1
 H2   NC   NC
 H3   VSS   GND
 H4   GW#   INBUF
 H5   VSS   GND
 H6   DQA5   Progbuf1
 H7   NC   NC
 J1   VDDQ   POWER
 J2   VDD   POWER
 J3   NC   NC
 J4   VDD   POWER
 J5   NC   NC
 J6   VDD   POWER
 J7   VDDQ   POWER
 K1   NC   NC
 K2   DQB5   Progbuf1
 K3   VSS   GND
 K4   CK   INBUF
 K5   VSS   GND
 K6   NC   NC
 K7   DQA4   Progbuf1
 L1   DQB6   Progbuf1
 L2   NC   NC
 L3   NC   NC
 L4   NC   NC
 L5   BA#   INBUF
 L6   DQA3   Progbuf1
 L7   NC   NC
 M1   VDDQ   POWER
 M2   DQB7   Progbuf1
 M3   VSS   GND
 M4   BW#   INBUF
 M5   VSS   GND
 M6   NC   NC
 M7   VDDQ   POWER
 N1   DQB8   Progbuf1
 N2   NC   NC
 N3   VSS   GND
 N4   A1   INBUF
 N5   VSS   GND
 N6   DQA2   Progbuf1
 N7   NC   NC
 P1   NC   NC
 P2   DQB9   Progbuf1
 P3   VSS   GND
 P4   A0   INBUF
 P5   VSS   GND
 P6   NC   NC
 P7   DQA1   Progbuf1
 R1   NC   NC
 R2   A2   INBUF
 R3   LBO#   INBUF
 R4   VDD   POWER
 R5   FT#   INBUF
 R6   A13   INBUF
 R7   NC   NC
 T1   NC   NC
 T2   A10   INBUF
 T3   A11   INBUF
 T4   NC   NC
 T5   A12   INBUF
 T6   A18   INBUF
 T7   ZZ   INBUF
 U1   VDDQ   POWER
 U2   TMS   INBUF
 U3   TDI   INBUF
 U4   TCK   INBUF
 U5   TDO   Progbuf2
 U6   NC   NC
 U7   VDDQ   POWER
[Component]   GS881E36CT
[Manufacturer]   gsi technology
[Package]
| variable   typ   min   max
R_pkg   0.2   0.1   0.5
L_pkg   4nH   2nH   6nH
C_pkg   1.5pF   1pF   2pF
[Pin]   signal_name model_name  R_pin   L_pin   C_pin
 1   DQC9   Progbuf1
 2   DQC8   Progbuf1
 3   DQC7   Progbuf1
 4   VDDQ   POWER
 5   VSS   GND
 6   DQC6   Progbuf1
 7   DQC5   Progbuf1
 8   DQC4   Progbuf1
 9   DQC3   Progbuf1
 10   VSS   GND
 11   VDDQ   POWER
 12   DQC2   Progbuf1
 13   DQC1   Progbuf1
 14   FT#   INBUF
 15   VDD   POWER
 16   NC   Progbuf1
 17   VSS   GND
 18   DQD1   Progbuf1
 19   DQD2   Progbuf1
 20   VDDQ   POWER
 21   VSS   GND
 22   DQD3   Progbuf1
 23   DQD4   Progbuf1
 24   DQD5   Progbuf1
 25   DQD6   Progbuf1
 26   VSS   GND
 27   VDDQ   POWER
 28   DQD7   Progbuf1
 29   DQD8   Progbuf1
 30   DQD9   Progbuf1
 31   LBO#   INBUF
 32   A5   INBUF
 33   A4   INBUF
 34   A3   INBUF
 35   A2   INBUF
 36   A1   INBUF
 37   A0   INBUF
 38   TMS   INBUF
 39   TDI   INBUF
 40   VSS   GND
 41   VDD   POWER
 42   TDO   Progbuf2
 43   TCK   INBUF
 44   A10   INBUF
 45   A11   INBUF
 46   A12   INBUF
 47   A13   INBUF
 48   A14   INBUF
 49   A15   INBUF
 50   A16   INBUF
 51   DQA9   Progbuf1
 52   DQA8   Progbuf1
 53   DQA7   Progbuf1
 54   VDDQ   POWER
 55   VSS   GND
 56   DQA6   Progbuf1
 57   DQA5   Progbuf1
 58   DQA4   Progbuf1
 59   DQA3   Progbuf1
 60   VSS   GND
 61   VDDQ   POWER
 62   DQA2   Progbuf1
 63   DQA1   Progbuf1
 64   ZZ   INBUF
 65   VDD   POWER
 66   NC   NC
 67   VSS   GND
 68   DQB1   Progbuf1
 69   DQB2   Progbuf1
 70   VDDQ   POWER
 71   VSS   GND
 72   DQB3   Progbuf1
 73   DQB4   Progbuf1
 74   DQB5   Progbuf1
 75   DQB6   Progbuf1
 76   VSS   GND
 77   VDDQ   POWER
 78   DQB7   Progbuf1
 79   DQB8   Progbuf1
 80   DQB9   Progbuf1
 81   A9   INBUF
 82   A8   INBUF
 83   ADV#   INBUF
 84   ADSP#   INBUF
 85   ADSC#   INBUF
 86   G#   INBUF
 87   BW#   INBUF
 88   GW#   INBUF
 89   CK   INBUF
 90   VSS   GND
 91   VDD   POWER
 92   A17   INBUF
 93   BA#   INBUF
 94   BB#   INBUF
 95   BC#   INBUF
 96   BD#   INBUF
 97   NC   NC
 98   E1#   INBUF
 99   A7   INBUF
 100   A6   INBUF
[Component]   GS881E36CD
[Manufacturer]   gsi technology
[Package]
| variable   typ   min   max
R_pkg   0.2   0.1   0.5
L_pkg   4nH   2nH   6nH
C_pkg   1.5pF   1pF   2pF
[Pin]   signal_name model_name  R_pin   L_pin   C_pin
 A1   NC   NC
 A2   A14   INBUF
 A3   E1#   INBUF
 A4   BC#   INBUF
 A5   BB#   INBUF
 A6   E3#   INBUF
 A7   BW#   INBUF
 A8   ADSC#   INBUF
 A9   ADV#   INBUF
 A10   A13   INBUF
 A11   NC   NC
 B1   NC   NC
 B2   A16   INBUF
 B3   E2   INBUF
 B4   BD#   INBUF
 B5   BA#   INBUF
 B6   CK   INBUF
 B7   GW#   INBUF
 B8   G#   INBUF
 B9   ADSP   INBUF
 B10   A15   INBUF
 B11   NC   NC
 C1   DQPC   Progbuf1
 C2   NC   NC
 C3   VDDQ   POWER
 C4   VSS   GND
 C5   VSS   GND
 C6   VSS   GND
 C7   VSS   GND
 C8   VSS   GND
 C9   VDDQ   POWER
 C10   NC   NC
 C11   DQPB   Progbuf1
 D1   DQC8   Progbuf1
 D2   DQC4   Progbuf1
 D3   VDDQ   POWER
 D4   VDD   POWER
 D5   VSS   GND
 D6   VSS   GND
 D7   VSS   GND
 D8   VDD   POWER
 D9   VDDQ   POWER
 D10   DQB4   Progbuf1
 D11   DQB8   Progbuf1
 E1   DQC7   Progbuf1
 E2   DQC3   Progbuf1
 E3   VDDQ   POWER
 E4   VDD   POWER
 E5   VSS   GND
 E6   VSS   GND
 E7   VSS   GND
 E8   VDD   POWER
 E9   VDDQ   POWER
 E10   DQB3   Progbuf1
 E11   DQB7   Progbuf1
 F1   DQC6   Progbuf1
 F2   DQC2   Progbuf1
 F3   VDDQ   POWER
 F4   VDD   POWER
 F5   VSS   GND
 F6   VSS   GND
 F7   VSS   GND
 F8   VDD   POWER
 F9   VDDQ   POWER
 F10   DQB2   Progbuf1
 F11   DQB6   Progbuf1
 G1   DQC5   Progbuf1
 G2   DQC1   Progbuf1
 G3   VDDQ   POWER
 G4   VDD   POWER
 G5   VSS   GND
 G6   VSS   GND
 G7   VSS   GND
 G8   VDD   POWER
 G9   VDDQ   POWER
 G10   DQB1   Progbuf1
 G11   DQB5   Progbuf1
 H1   FT#   INBUF
 H2   MCL   INBUF
 H3   NC   NC
 H4   VDD   POWER
 H5   VSS   GND
 H6   VSS   GND
 H7   VSS   GND
 H8   VDD   POWER
 H9   NC   NC
 H10   NC   NC
 H11   ZZ   INBUF
 J1   DQD5   Progbuf1
 J2   DQD1   Progbuf1
 J3   VDDQ   POWER
 J4   VDD   POWER
 J5   VSS   GND
 J6   VSS   GND
 J7   VSS   GND
 J8   VDD   POWER
 J9   VDDQ   POWER
 J10   DQA1   Progbuf1
 J11   DQA5   Progbuf1
 K1   DQD6   Progbuf1
 K2   DQD2   Progbuf1
 K3   VDDQ   POWER
 K4   VDD   POWER
 K5   VSS   GND
 K6   VSS   GND
 K7   VSS   GND
 K8   VDD   POWER
 K9   VDDQ   POWER
 K10   DQA2   Progbuf1
 K11   DQA6   Progbuf1
 L1   DQD7   Progbuf1
 L2   DQD3   Progbuf1
 L3   VDDQ   POWER
 L4   VDD   POWER
 L5   VSS   GND
 L6   VSS   GND
 L7   VSS   GND
 L8   VDD   POWER
 L9   VDDQ   POWER
 L10   DQA3   Progbuf1
 L11   DQA7   Progbuf1
 M1   DQD8   Progbuf1
 M2   DQD4   Progbuf1
 M3   VDDQ   POWER
 M4   VDD   POWER
 M5   VSS   GND
 M6   VSS   GND
 M7   VSS   GND
 M8   VDD   POWER
 M9   VDDQ   POWER
 M10   DQA4   Progbuf1
 M11   DQA8   Progbuf1
 N1   DQPD   Progbuf1
 N2   NC   NC
 N3   VDDQ   POWER
 N4   VSS   GND
 N5   NC   NC
 N6   NC   NC
 N7   NC   NC
 N8   VSS   GND
 N9   VDDQ   POWER
 N10   NC   NC
 N11   DQPA   Progbuf1
 P1   NC   NC
 P2   NC   NC
 P3   A6   INBUF
 P4   A5   INBUF
 P5   TDI   INBUF
 P6   A1   INBUF
 P7   TDO   Progbuf2
 P8   A4   INBUF
 P9   A3   INBUF
 P10   A2   INBUF
 P11   A17   INBUF
 R1   LBO#   INBUF
 R2   NC   NC
 R3   A12   INBUF
 R4   A11   INBUF
 R5   TMS   INBUF
 R6   A0   INBUF
 R7   TCK   INBUF
 R8   A10   INBUF
 R9   A9   INBUF
 R10   A8   INBUF
 R11   A7   INBUF
[Component]   GS88118CT
[Manufacturer]   gsi technology
[Package]
| variable   typ   min   max
R_pkg   0.2   0.1   0.5
L_pkg   4nH   2nH   6nH
C_pkg   1.5pF   1pF   2pF
[Pin]   signal_name model_name  R_pin   L_pin   C_pin
 1   NC   NC
 2   NC   NC
 3   NC   NC
 4   VDDQ   POWER
 5   VSS   GND
 6   NC   NC
 7   NC   NC
 8   DQB1   Progbuf1
 9   DQB2   Progbuf1
 10   VSS   GND
 11   VDDQ   POWER
 12   DQB3   Progbuf1
 13   DQB4   Progbuf1
 14   FT#   INBUF
 15   VDD   POWER
 16   NC   NC
 17   VSS   GND
 18   DQB5   Progbuf1
 19   DQB6   Progbuf1
 20   VDDQ   POWER
 21   VSS   GND
 22   DQB7   Progbuf1
 23   DQB8   Progbuf1
 24   DQB9   Progbuf1
 25   NC   NC
 26   VSS   GND
 27   VDDQ   POWER
 28   NC   NC
 29   NC   NC
 30   NC   NC
 31   LBO#   INBUF
 32   A5   INBUF
 33   A4   INBUF
 34   A3   INBUF
 35   A2   INBUF
 36   A1   INBUF
 37   A0   INBUF
 38   TMS   INBUF
 39   TDI   INBUF
 40   VSS   GND
 41   VDD   POWER
 42   TDO   Progbuf2
 43   TCK   INBUF
 44   A10   INBUF
 45   A11   INBUF
 46   A12   INBUF
 47   A13   INBUF
 48   A14   INBUF
 49   A15   INBUF
 50   A16   INBUF
 51   NC   NC
 52   NC   NC
 53   NC   NC
 54   VDDQ   POWER
 55   VSS   GND
 56   DQA6   Progbuf1
 57   NC   NC
 58   DQA1   Progbuf1
 59   DQA2   Progbuf1
 60   VSS   GND
 61   VDDQ   POWER
 62   DQA3   Progbuf1
 63   DQA4   Progbuf1
 64   ZZ   INBUF
 65   VDD   POWER
 66   NC   NC
 67   VSS   GND
 68   DQA5   Progbuf1
 69   DQA6   Progbuf1
 70   VDDQ   POWER
 71   VSS   GND
 72   DQA7   Progbuf1
 73   DQA8   Progbuf1
 74   DQA9   Progbuf1
 75   NC   NC
 76   VSS   GND
 77   VDDQ   POWER
 78   NC   NC
 79   NC   NC
 80   A18   INBUF
 81   A9   INBUF
 82   A8   INBUF
 83   ADV#   INBUF
 84   ADSP#   INBUF
 85   ADSC#   INBUF
 86   G#   INBUF
 87   BW#   INBUF
 88   GW#   INBUF
 89   CK   INBUF
 90   VSS   GND
 91   VDD   POWER
 92   A17   INBUF
 93   BA#   INBUF
 94   BB#   INBUF
 95   NC   NC
 96   NC   NC
 97   NC   NC
 98   E1#   INBUF
 99   A7   INBUF
 100   A6   INBUF
[Component]   GS88118CD
[Manufacturer]   gsi technology
[Package]
| variable   typ   min   max
R_pkg   0.2   0.1   0.5
L_pkg   3nH   1nH   5nH
C_pkg   1.5pF   1pF   3pF
[Pin]   signal_name model_name  R_pin   L_pin   C_pin
 A1   VDDQ   POWER
 A2   A6   INBUF
 A3   A7   INBUF
 A4   ADSP#   INBUF
 A5   A8   INBUF
 A6   A9   INBUF
 A7   VDDQ   POWER
 B1   NC   NC
 B2   NC   NC
 B3   A4   INBUF
 B4   ADSC#   INBUF
 B5   A15   INBUF
 B6   A17   INBUF
 B7   NC   NC
 C1   NC   NC
 C2   A5   INBUF
 C3   A3   INBUF
 C4   VDD   POWER
 C5   A14   INBUF
 C6   A16   INBUF
 C7   NC   NC
 D1   DQB1   Progbuf1
 D2   NC   NC
 D3   VSS   GND
 D4   NC   NC
 D5   VSS   GND
 D6   DQA9   Progbuf1
 D7   NC   NC
 E1   NC   NC
 E2   DQB2   Progbuf1
 E3   VSS   GND
 E4   E1#   INBUF
 E5   VSS   GND
 E6   NC   NC
 E7   DQA8   Progbuf1
 F1   VDDQ   POWER
 F2   NC   NC
 F3   VSS   GND
 F4   G#   INBUF
 F5   VSS   GND
 F6   DQA7   Progbuf1
 F7   VDDQ   POWER
 G1   NC   NC
 G2   DQB3   Progbuf1
 G3   BB#   INBUF
 G4   ADV#   INBUF
 G5   NC   NC
 G6   NC   NC
 G7   DQA6   Progbuf1
 H1   DQB4   Progbuf1
 H2   NC   NC
 H3   VSS   GND
 H4   GW#   INBUF
 H5   VSS   GND
 H6   DQA5   Progbuf1
 H7   NC   NC
 J1   VDDQ   POWER
 J2   VDD   POWER
 J3   NC   NC
 J4   VDD   POWER
 J5   NC   NC
 J6   VDD   POWER
 J7   VDDQ   POWER
 K1   NC   NC
 K2   DQB5   Progbuf1
 K3   VSS   GND
 K4   CK   INBUF
 K5   VSS   GND
 K6   NC   NC
 K7   DQA4   Progbuf1
 L1   DQB6   Progbuf1
 L2   NC   NC
 L3   NC   NC
 L4   NC   NC
 L5   BA#   INBUF
 L6   DQA3   Progbuf1
 L7   NC   NC
 M1   VDDQ   POWER
 M2   DQB7   Progbuf1
 M3   VSS   GND
 M4   BW#   INBUF
 M5   VSS   GND
 M6   NC   NC
 M7   VDDQ   POWER
 N1   DQB8   Progbuf1
 N2   NC   NC
 N3   VSS   GND
 N4   A1   INBUF
 N5   VSS   GND
 N6   DQA2   Progbuf1
 N7   NC   NC
 P1   NC   NC
 P2   DQB9   Progbuf1
 P3   VSS   GND
 P4   A0   INBUF
 P5   VSS   GND
 P6   NC   NC
 P7   DQA1   Progbuf1
 R1   NC   NC
 R2   A2   INBUF
 R3   LBO#   INBUF
 R4   VDD   POWER
 R5   FT#   INBUF
 R6   A13   INBUF
 R7   NC   NC
 T1   NC   NC
 T2   A10   INBUF
 T3   A11   INBUF
 T4   NC   NC
 T5   A12   INBUF
 T6   A18   INBUF
 T7   ZZ   INBUF
 U1   VDDQ   POWER
 U2   TMS   INBUF
 U3   TDI   INBUF
 U4   TCK   INBUF
 U5   TDO   Progbuf2
 U6   NC   NC
 U7   VDDQ   POWER
[Component]   GS88136CT
[Manufacturer]   gsi technology
[Package]
| variable   typ   min   max
R_pkg   0.2   0.1   0.5
L_pkg   4nH   2nH   6nH
C_pkg   1.5pF   1pF   2pF
[Pin]   signal_name model_name  R_pin   L_pin   C_pin
 1   DQC9   Progbuf1
 2   DQC8   Progbuf1
 3   DQC7   Progbuf1
 4   VDDQ   POWER
 5   VSS   GND
 6   DQC6   Progbuf1
 7   DQC5   Progbuf1
 8   DQC4   Progbuf1
 9   DQC3   Progbuf1
 10   VSS   GND
 11   VDDQ   POWER
 12   DQC2   Progbuf1
 13   DQC1   Progbuf1
 14   FT#   INBUF
 15   VDD   POWER
 16   NC   Progbuf1
 17   VSS   GND
 18   DQD1   Progbuf1
 19   DQD2   Progbuf1
 20   VDDQ   POWER
 21   VSS   GND
 22   DQD3   Progbuf1
 23   DQD4   Progbuf1
 24   DQD5   Progbuf1
 25   DQD6   Progbuf1
 26   VSS   GND
 27   VDDQ   POWER
 28   DQD7   Progbuf1
 29   DQD8   Progbuf1
 30   DQD9   Progbuf1
 31   LBO#   INBUF
 32   A5   INBUF
 33   A4   INBUF
 34   A3   INBUF
 35   A2   INBUF
 36   A1   INBUF
 37   A0   INBUF
 38   TMS   INBUF
 39   TDI   INBUF
 40   VSS   GND
 41   VDD   POWER
 42   TDO   Progbuf2
 43   TCK   INBUF
 44   A10   INBUF
 45   A11   INBUF
 46   A12   INBUF
 47   A13   INBUF
 48   A14   INBUF
 49   A15   INBUF
 50   A16   INBUF
 51   DQA9   Progbuf1
 52   DQA8   Progbuf1
 53   DQA7   Progbuf1
 54   VDDQ   POWER
 55   VSS   GND
 56   DQA6   Progbuf1
 57   DQA5   Progbuf1
 58   DQA4   Progbuf1
 59   DQA3   Progbuf1
 60   VSS   GND
 61   VDDQ   POWER
 62   DQA2   Progbuf1
 63   DQA1   Progbuf1
 64   ZZ   INBUF
 65   VDD   POWER
 66   NC   NC
 67   VSS   GND
 68   DQB1   Progbuf1
 69   DQB2   Progbuf1
 70   VDDQ   POWER
 71   VSS   GND
 72   DQB3   Progbuf1
 73   DQB4   Progbuf1
 74   DQB5   Progbuf1
 75   DQB6   Progbuf1
 76   VSS   GND
 77   VDDQ   POWER
 78   DQB7   Progbuf1
 79   DQB8   Progbuf1
 80   DQB9   Progbuf1
 81   A9   INBUF
 82   A8   INBUF
 83   ADV#   INBUF
 84   ADSP#   INBUF
 85   ADSC#   INBUF
 86   G#   INBUF
 87   BW#   INBUF
 88   GW#   INBUF
 89   CK   INBUF
 90   VSS   GND
 91   VDD   POWER
 92   A17   INBUF
 93   BA#   INBUF
 94   BB#   INBUF
 95   BC#   INBUF
 96   BD#   INBUF
 97   NC   NC
 98   E1#   INBUF
 99   A7   INBUF
 100   A6   INBUF
[Component]   GS88136CD
[Manufacturer]   gsi technology
[Package]
| variable   typ   min   max
R_pkg   0.2   0.1   0.5
L_pkg   4nH   2nH   6nH
C_pkg   1.5pF   1pF   2pF
[Pin]   signal_name model_name  R_pin   L_pin   C_pin
 A1   NC   NC
 A2   A14   INBUF
 A3   E1#   INBUF
 A4   BC#   INBUF
 A5   BB#   INBUF
 A6   E3#   INBUF
 A7   BW#   INBUF
 A8   ADSC#   INBUF
 A9   ADV#   INBUF
 A10   A13   INBUF
 A11   NC   NC
 B1   NC   NC
 B2   A16   INBUF
 B3   E2   INBUF
 B4   BD#   INBUF
 B5   BA#   INBUF
 B6   CK   INBUF
 B7   GW#   INBUF
 B8   G#   INBUF
 B9   ADSP   INBUF
 B10   A15   INBUF
 B11   NC   NC
 C1   DQPC   Progbuf1
 C2   NC   NC
 C3   VDDQ   POWER
 C4   VSS   GND
 C5   VSS   GND
 C6   VSS   GND
 C7   VSS   GND
 C8   VSS   GND
 C9   VDDQ   POWER
 C10   NC   NC
 C11   DQPB   Progbuf1
 D1   DQC8   Progbuf1
 D2   DQC4   Progbuf1
 D3   VDDQ   POWER
 D4   VDD   POWER
 D5   VSS   GND
 D6   VSS   GND
 D7   VSS   GND
 D8   VDD   POWER
 D9   VDDQ   POWER
 D10   DQB4   Progbuf1
 D11   DQB8   Progbuf1
 E1   DQC7   Progbuf1
 E2   DQC3   Progbuf1
 E3   VDDQ   POWER
 E4   VDD   POWER
 E5   VSS   GND
 E6   VSS   GND
 E7   VSS   GND
 E8   VDD   POWER
 E9   VDDQ   POWER
 E10   DQB3   Progbuf1
 E11   DQB7   Progbuf1
 F1   DQC6   Progbuf1
 F2   DQC2   Progbuf1
 F3   VDDQ   POWER
 F4   VDD   POWER
 F5   VSS   GND
 F6   VSS   GND
 F7   VSS   GND
 F8   VDD   POWER
 F9   VDDQ   POWER
 F10   DQB2   Progbuf1
 F11   DQB6   Progbuf1
 G1   DQC5   Progbuf1
 G2   DQC1   Progbuf1
 G3   VDDQ   POWER
 G4   VDD   POWER
 G5   VSS   GND
 G6   VSS   GND
 G7   VSS   GND
 G8   VDD   POWER
 G9   VDDQ   POWER
 G10   DQB1   Progbuf1
 G11   DQB5   Progbuf1
 H1   FT#   INBUF
 H2   MCL   INBUF
 H3   NC   NC
 H4   VDD   POWER
 H5   VSS   GND
 H6   VSS   GND
 H7   VSS   GND
 H8   VDD   POWER
 H9   NC   NC
 H10   NC   NC
 H11   ZZ   INBUF
 J1   DQD5   Progbuf1
 J2   DQD1   Progbuf1
 J3   VDDQ   POWER
 J4   VDD   POWER
 J5   VSS   GND
 J6   VSS   GND
 J7   VSS   GND
 J8   VDD   POWER
 J9   VDDQ   POWER
 J10   DQA1   Progbuf1
 J11   DQA5   Progbuf1
 K1   DQD6   Progbuf1
 K2   DQD2   Progbuf1
 K3   VDDQ   POWER
 K4   VDD   POWER
 K5   VSS   GND
 K6   VSS   GND
 K7   VSS   GND
 K8   VDD   POWER
 K9   VDDQ   POWER
 K10   DQA2   Progbuf1
 K11   DQA6   Progbuf1
 L1   DQD7   Progbuf1
 L2   DQD3   Progbuf1
 L3   VDDQ   POWER
 L4   VDD   POWER
 L5   VSS   GND
 L6   VSS   GND
 L7   VSS   GND
 L8   VDD   POWER
 L9   VDDQ   POWER
 L10   DQA3   Progbuf1
 L11   DQA7   Progbuf1
 M1   DQD8   Progbuf1
 M2   DQD4   Progbuf1
 M3   VDDQ   POWER
 M4   VDD   POWER
 M5   VSS   GND
 M6   VSS   GND
 M7   VSS   GND
 M8   VDD   POWER
 M9   VDDQ   POWER
 M10   DQA4   Progbuf1
 M11   DQA8   Progbuf1
 N1   DQPD   Progbuf1
 N2   NC   NC
 N3   VDDQ   POWER
 N4   VSS   GND
 N5   NC   NC
 N6   NC   NC
 N7   NC   NC
 N8   VSS   GND
 N9   VDDQ   POWER
 N10   NC   NC
 N11   DQPA   Progbuf1
 P1   NC   NC
 P2   NC   NC
 P3   A6   INBUF
 P4   A5   INBUF
 P5   TDI   INBUF
 P6   A1   INBUF
 P7   TDO   Progbuf2
 P8   A4   INBUF
 P9   A3   INBUF
 P10   A2   INBUF
 P11   A17   INBUF
 R1   LBO#   INBUF
 R2   NC   NC
 R3   A12   INBUF
 R4   A11   INBUF
 R5   TMS   INBUF
 R6   A0   INBUF
 R7   TCK   INBUF
 R8   A10   INBUF
 R9   A9   INBUF
 R10   A8   INBUF
 R11   A7   INBUF
[Component]   GS88218CB
[Manufacturer]   gsi technology
[Package]
| variable   typ   min   max
R_pkg   0.2   0.1   0.5
L_pkg   3nH   1nH   5nH
C_pkg   1.5pF   1pF   3pF
[Pin]   signal_name model_name  R_pin   L_pin   C_pin
 1A   VDDQ   POWER
 1B   NC   NC
 1C   NC   NC
 1D   DQB1   Progbuf1
 1E   NC   NC
 1F   VDDQ   POWER
 1G   NC   NC
 1H   DQB4   Progbuf1
 1J   VDDQ   POWER
 1K   NC   NC
 1L   DQB6   Progbuf1
 1M   VDDQ   POWER
 1N   DQB8   Progbuf1
 1P   NC   NC
 1R   NC   NC
 1T   NC   NC
 1U   VDDQ   POWER
 2A   A6   INBUF
 2B   A18   INBUF
 2C   A5   INBUF
 2D   NC   NC
 2E   DQB2   Progbuf1
 2F   NC   NC
 2G   DQB3   Progbuf1
 2H   NC   NC
 2J   VDD   POWER
 2K   DQB5   Progbuf1
 2L   NC   NC
 2M   DQB7   Progbuf1
 2N   NC   NC
 2P   DQB9   Progbuf1
 2R   A2   INBUF
 2T   A10   INBUF
 2U   TMS   INBUF
 3A   A7   INBUF
 3B   A4   INBUF
 3C   A3   INBUF
 3D   VSS   GND
 3E   VSS   GND
 3F   VSS   GND
 3G   BB#   INBUF
 3H   VSS   GND
 3J   DP   INBUF
 3K   VSS   GND
 3L   NC   NC
 3M   VSS   GND
 3N   VSS   GND
 3P   VSS   GND
 3R   LBO#   INBUF
 3T   A11   INBUF
 3U   TDI   INBUF
 4A   ADSP#   INBUF
 4B   ADSC#   INBUF
 4C   VDD   POWER
 4D   ZQ   INBUF
 4E   E1#   INBUF
 4F   G#   INBUF
 4G   ADV#   INBUF
 4H   GW#   INBUF
 4J   VDD   POWER
 4K   CK   INBUF
 4L   SCD   INBUF
 4M   BW#   INBUF
 4N   A1   INBUF
 4P   A0   INBUF
 4R   VDD   POWER
 4T   NC   NC
 4U   TCK   INBUF
 5A   A8   INBUF
 5B   A15   INBUF
 5C   A14   INBUF
 5D   VSS   GND
 5E   VSS   GND
 5F   VSS   GND
 5G   NC   NC
 5H   VSS   GND
 5J   NC   NC
 5K   VSS   GND
 5L   BA#   INBUF
 5M   VSS   GND
 5N   VSS   GND
 5P   VSS   GND
 5R   FT#   INBUF
 5T   A12   INBUF
 5U   TDO   Progbuf2
 6A   A9   INBUF
 6B   A17   INBUF
 6C   A16   INBUF
 6D   DQA9   Progbuf1
 6E   NC   NC
 6F   DQA7   Progbuf1
 6G   NC   NC
 6H   DQA5   Progbuf1
 6J   VDD   POWER
 6K   NC   NC
 6L   DQA3   Progbuf1
 6M   NC   NC
 6N   DQA2   Progbuf1
 6P   NC   NC
 6R   A13   INBUF
 6T   A19   INBUF
 6U   NC   NC
 7A   VDDQ   POWER
 7B   NC   NC
 7C   NC   NC
 7D   NC   NC
 7E   DQA8   Progbuf1
 7F   VDDQ   POWER
 7G   DQA6   Progbuf1
 7H   NC   NC
 7J   VDDQ   POWER
 7K   DQA4   Progbuf1
 7L   NC   NC
 7M   VDDQ   POWER
 7N   NC   NC
 7P   DQA1   Progbuf1
 7R   PE#   INBUF
 7T   ZZ   INBUF
 7U   VDDQ   POWER
[Component]   GS88219CB
[Manufacturer]   gsi technology
[Package]
| variable   typ   min   max
R_pkg   0.2   0.1   0.5
L_pkg   3nH   1nH   5nH
C_pkg   1.5pF   1pF   3pF
[Pin]   signal_name model_name  R_pin   L_pin   C_pin
 1A   VDDQ   POWER
 1B   NC   NC
 1C   NC   NC
 1D   DQB1   Progbuf1
 1E   NC   NC
 1F   VDDQ   POWER
 1G   NC   NC
 1H   DQB4   Progbuf1
 1J   VDDQ   POWER
 1K   NC   NC
 1L   DQB6   Progbuf1
 1M   VDDQ   POWER
 1N   DQB8   Progbuf1
 1P   NC   NC
 1R   NC   NC
 1T   NC   NC
 1U   VDDQ   POWER
 2A   A6   INBUF
 2B   A18   INBUF
 2C   A5   INBUF
 2D   NC   NC
 2E   DQB2   Progbuf1
 2F   NC   NC
 2G   DQB3   Progbuf1
 2H   NC   NC
 2J   VDD   POWER
 2K   DQB5   Progbuf1
 2L   NC   NC
 2M   DQB7   Progbuf1
 2N   NC   NC
 2P   DQB9   Progbuf1
 2R   A2   INBUF
 2T   A10   INBUF
 2U   TMS   INBUF
 3A   A7   INBUF
 3B   A4   INBUF
 3C   A3   INBUF
 3D   VSS   GND
 3E   VSS   GND
 3F   VSS   GND
 3G   BB#   INBUF
 3H   VSS   GND
 3J   DP   INBUF
 3K   VSS   GND
 3L   NC   NC
 3M   VSS   GND
 3N   VSS   GND
 3P   VSS   GND
 3R   LBO#   INBUF
 3T   A11   INBUF
 3U   TDI   INBUF
 4A   ADSP#   INBUF
 4B   ADSC#   INBUF
 4C   VDD   POWER
 4D   ZQ   INBUF
 4E   E1#   INBUF
 4F   G#   INBUF
 4G   ADV#   INBUF
 4H   GW#   INBUF
 4J   VDD   POWER
 4K   CK   INBUF
 4L   SCD   INBUF
 4M   BW#   INBUF
 4N   A1   INBUF
 4P   A0   INBUF
 4R   VDD   POWER
 4T   NC   NC
 4U   TCK   INBUF
 5A   A8   INBUF
 5B   A15   INBUF
 5C   A14   INBUF
 5D   VSS   GND
 5E   VSS   GND
 5F   VSS   GND
 5G   NC   NC
 5H   VSS   GND
 5J   NC   NC
 5K   VSS   GND
 5L   BA#   INBUF
 5M   VSS   GND
 5N   VSS   GND
 5P   VSS   GND
 5R   FT#   INBUF
 5T   A12   INBUF
 5U   TDO   Progbuf2
 6A   A9   INBUF
 6B   A17   INBUF
 6C   A16   INBUF
 6D   DQA9   Progbuf1
 6E   NC   NC
 6F   DQA7   Progbuf1
 6G   NC   NC
 6H   DQA5   Progbuf1
 6J   VDD   POWER
 6K   NC   NC
 6L   DQA3   Progbuf1
 6M   NC   NC
 6N   DQA2   Progbuf1
 6P   NC   NC
 6R   A13   INBUF
 6T   A19   INBUF
 6U   NC   NC
 7A   VDDQ   POWER
 7B   NC   NC
 7C   NC   NC
 7D   NC   NC
 7E   DQA8   Progbuf1
 7F   VDDQ   POWER
 7G   DQA6   Progbuf1
 7H   NC   NC
 7J   VDDQ   POWER
 7K   DQA4   Progbuf1
 7L   NC   NC
 7M   VDDQ   POWER
 7N   NC   NC
 7P   DQA1   Progbuf1
 7R   PE#   INBUF
 7T   ZZ   INBUF
 7U   VDDQ   POWER
[Component]   GS88218CD
[Manufacturer]   gsi technology
[Package]
| variable   typ   min   max
R_pkg   0.2   0.1   0.5
L_pkg   3nH   1nH   5nH
C_pkg   1.5pF   1pF   3pF
[Pin]   signal_name model_name  R_pin   L_pin   C_pin
 A1   NC   NC
 A2   A14   INBUF
 A3   E1#   INBUF
 A4   BB#   INBUF
 A5   NC   NC
 A6   E3#   INBUF
 A7   BW#   INBUF
 A8   ADSC#   INBUF
 A9   ADV#   INBUF
 A10   A13   INBUF
 A11   A18   INBUF
 B1   NC   NC
 B2   A16   INBUF
 B3   E2   INBUF
 B4   NC   NC
 B5   BA#   INBUF
 B6   CK   INBUF
 B7   GW#   INBUF
 B8   G#   INBUF
 B9   ADSP   INBUF
 B10   A15   INBUF
 B11   NC   NC
 C1   NC   NC
 C2   NC   NC
 C3   VDDQ   POWER
 C4   VSS   GND
 C5   VSS   GND
 C6   VSS   GND
 C7   VSS   GND
 C8   VSS   GND
 C9   VDDQ   POWER
 C10   NC   NC
 C11   DQPA   Progbuf1
 D1   NC   NC
 D2   DQB1   Progbuf1
 D3   VDDQ   POWER
 D4   VDD   POWER
 D5   VSS   GND
 D6   VSS   GND
 D7   VSS   GND
 D8   VDD   POWER
 D9   VDDQ   POWER
 D10   NC   NC
 D11   DQA8   Progbuf1
 E1   NC   NC
 E2   DQB2   Progbuf1
 E3   VDDQ   POWER
 E4   VDD   POWER
 E5   VSS   GND
 E6   VSS   GND
 E7   VSS   GND
 E8   VDD   POWER
 E9   VDDQ   POWER
 E10   NC   NC
 E11   DQA7   Progbuf1
 F1   NC   NC
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| Models and submodels in the file (18): VIO_1Ldriver (I/O), VIO_1Hdriver (I/O), VIO_2Ldriver (I/O), VIO_2Hdriver (I/O), VIO_3Ldriver (I/O), VIO_3Hdriver (I/O), VIO_4Ldriver (I/O), VIO_4Hdriver (I/O), VIO_5Ldriver (I/O), VIO_5Hdriver (I/O), TDO_1driver (3-state), TDO_2driver (3-state), TDO_3driver (3-state), TDO_4driver (3-state), TDO_5driver (3-state), INBUF_1.8 (Input), INBUF_2.5 (Input), INBUF_3.3 (Input)
